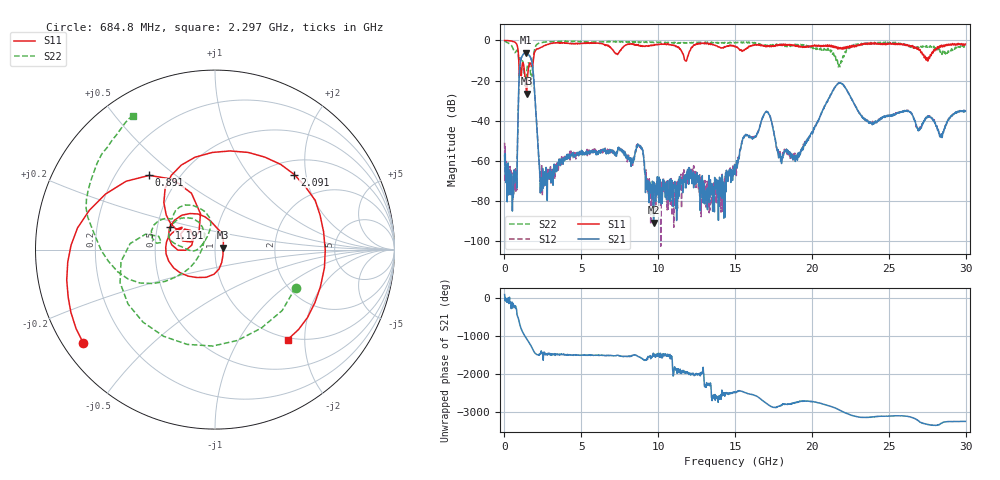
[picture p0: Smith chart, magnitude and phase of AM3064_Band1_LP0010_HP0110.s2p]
# Hz S DB R 50.0
!freq dBS11 angS11 dBS21 angS21 dBS12 angS12 dBS22 angS22
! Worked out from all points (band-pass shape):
!   1600 points, 10 MHz to 29.98 GHz, reference 50 ohm
!   highest |S21| = -6.08 dB at 1.397 GHz (marker M1); lowest = -90.8 dB at 9.701 GHz (marker M2)
!   |S21| within 3 dB of the highest: 1.083 GHz to 1.727 GHz (643.7 MHz wide, 45.8 % of centre)
!   lowest |S11| = -26.6 dB at 1.435 GHz (marker M3), VSWR 1.10, Z = 54.8 + j1.09 ohm
!   |S11| at or under -10 dB: 931.5 MHz to 1.878 GHz (946.6 MHz wide, 67.4 % of centre); 11.75 GHz to 11.84 GHz (89.88 MHz wide, 0.762 % of centre); 27.52052 GHz to 27.54952 GHz (28.99 MHz wide, 0.105 % of centre)
!   |S22| runs from -22.9 to -0.3 dB; largest |S21 - S12| = 0.0056
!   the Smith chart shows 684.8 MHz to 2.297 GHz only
!   S11 on the Smith chart (normalised r, x): 684.8 MHz: 0.06, -0.32; 891 MHz: 0.34, +0.41; 1.191 GHz: 0.58, +0.16; 2.091 GHz: 1.30, +1.72; 2.297 GHz: 0.96, -1.66
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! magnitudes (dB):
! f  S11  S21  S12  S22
! 10 MHz  0.0  -57.3  -50.9  -0.3
! 684.8 MHz  -0.9  -69.8  -74.3  -6.1
! 891 MHz  -5.2  -35.7  -35.7  -6.5
! 1.191 GHz  -11.0  -7.3  -7.3  -10.5
! 1.397 GHz  -21.3  -6.1  -6.1  -18.4
! 1.435 GHz  -26.6  -6.2  -6.1  -16.0
! 1.791 GHz  -13.1  -10.9  -10.9  -17.5
! 2.091 GHz  -4.3  -41.3  -41.4  -2.2
! 2.297 GHz  -3.8  -65.9  -67.2  -1.2
! 5.015 GHz  -1.5  -54.7  -55.8  -0.6
! 8.782 GHz  -2.7  -52.6  -53.0  -0.8
! 9.701 GHz  -2.5  -90.8  -72.2  -1.0
! 10 GHz  -2.0  -73.7  -72.4  -0.9
! 14.07 GHz  -3.7  -74.2  -81.0  -1.2
! 15 GHz  -3.1  -66.8  -64.3  -1.2
! 17.01 GHz  -3.2  -35.7  -35.6  -2.5
! 17.97 GHz  -2.5  -60.3  -58.4  -2.1
! 19.99 GHz  -3.0  -46.1  -45.9  -3.4
! 21.79 GHz  -4.0  -21.3  -21.0  -12.2
! 25 GHz  -1.4  -37.7  -37.2  -1.2
! 28.41 GHz  -2.4  -47.5  -46.5  -5.3
! 29.98 GHz  -1.8  -35.2  -35.1  -3.1
